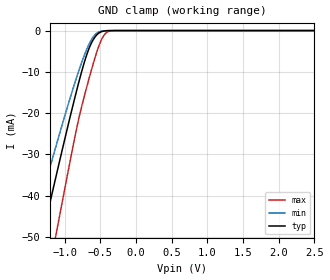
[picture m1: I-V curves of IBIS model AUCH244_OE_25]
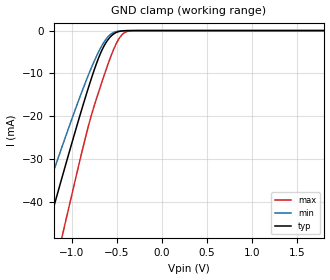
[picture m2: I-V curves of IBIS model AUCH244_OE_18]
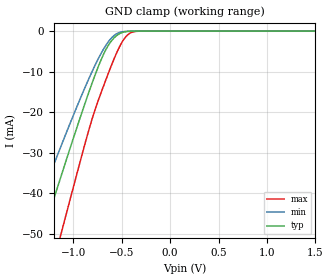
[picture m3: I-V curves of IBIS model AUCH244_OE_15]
| TEXAS INSTRUMENTS INCORPORATED
| Standard Linear and Logic Group
| IBIS Model of SN74AUCH244
| OCTAL BUFFER/DRIVER WITH 3-STATE OUTPUTS
| This file contains package information for the following:
|  QFN 20-pin (RGY) package as [Component] AUCH244_RGY
| This device can be powered at the following Vccs:
|  2.5 volt Vcc
|  1.8 volt Vcc
|  1.5 volt Vcc
|  1.2 volt Vcc
|  0.8 volt Vcc
| This file provides unique models under the [Model Selector] for each Vcc.
| For operation at a specific Vcc, select the appropriate model after each
| [Model Selector] keyword.
[IBIS Ver]   3.2
[Comment char]  |_char
[File Name]   sn74auch244.ibs
[File Rev]   1.1 | x_die
[Date]   October 17, 2002
[Source]   Data created from TI-SPICE simulations at TI-SLL.
[Notes]   The following is an IBIS list for the SN74AUCH244.
   Please contact sllibis@ti.com with questions and
   comments concerning SLL IBIS models.
   -The waveforms for the AUCH244_OUT Pullup and
   Pulldown are caused by the circuitry that helps reduce
   overshoot and undershoot in transmission lines (EMI).
   These waveforms are normal for this particular design.
   -Power-clamp data has been deleted since there is no
   power-clamp diode in the device.
   -Due to presence of bus hold at input, GND-clamp curves
   have non-monotonic warnings.
   -Due to the fact that the device is 5-V input/output
   tolerant, the pullup data has some non-monotonic warnings.
   -End point warning due to AC and DC mismatch.
[Disclaimer] Property of Texas Instruments Incorporated.  Unauthorized
   reproduction and/or distribution is strictly prohibited.
   This product is protected under copyright law.
   Created  2002, (C) Copyright  2002, Texas Instruments
   Incorporated, All Rights Reserved
   UNLESS THERE IS A SIGNED, WRITTEN AGREEMENT TO THE
   CONTRARY, TEXAS INSTRUMENTS (TI) IS PROVIDING THE IBIS
   MODELS  AND WITHOUT ANY WARRANTY, EXPRESSED OR
   IMPLIED.  TI assumes no liability for:
   1) the accuracy of the IBIS models provided to your
   company;
   2) the proper functioning of these IBIS Models in your
   design or for any resulting applications; or
   3) infringement of patents, copyrights or intellectual
   property rights resulting from your use of these IBIS
   models.
   TI provides IBIS Models as a service to our customers.
   You and your company shall not distribute, sell or give
   these models to anyone else without prior written
   permission from TI.
   TI reserves the right to make changes to our products or
   to discontinue any semiconductor product or service
   without notice, and advises our customers to obtain the
   latest version of relevant information to verify, before
   placing orders, that the information being relied on is
   current.
   Please be aware that your receipt and use of the IBIS
   information provided shall serve as acceptance of these
   terms and conditions.  If you do not accept these terms,
   you should return or destroy the IBIS models and any
   other accompanying information immediately.
| Component AUCH244_RGY 20-pin QFN
[Component]   AUCH244_RGY
[Manufacturer]   Texas Instruments, Inc.
[Package]
|   typ   min   max
R_pkg   0.046   0.035   0.058
L_pkg   1.131nH   0.880nH   1.396nH
C_pkg   0.165pF   0.142pF   0.175pF
[Pin]   signal_name   model_name   R_pin   L_pin   C_pin
1   1NOE   AUCH244_OE   0.053   1.289nH   0.142pF
2   1A1   AUCH244_IN   0.058   1.386nH   0.172pF
3   2Y4   AUCH244_OUT   0.046   1.111nH   0.173pF
4   1A2   AUCH244_IN   0.039   0.965nH   0.161pF
5   2Y3   AUCH244_OUT   0.035   0.881nH   0.165pF
6   1A3   AUCH244_IN   0.035   0.880nH   0.165pF
7   2Y2   AUCH244_OUT   0.039   0.961nH   0.161pF
8   1A4   AUCH244_IN   0.045   1.105nH   0.172pF
9   2Y1   AUCH244_OUT   0.058   1.386nH   0.172pF
10   GND   GND   0.056   1.352nH   0.159pF
11   2A1   AUCH244_IN   0.053   1.287nH   0.155pF
12   1Y4   AUCH244_OUT   0.058   1.396nH   0.172pF
13   2A2   AUCH244_IN   0.047   1.129nH   0.175pF
14   1Y3   AUCH244_OUT   0.040   0.976nH   0.164pF
15   2A3   AUCH244_IN   0.035   0.884nH   0.169pF
16   1Y2   AUCH244_OUT   0.035   0.881nH   0.168pF
17   2A4   AUCH244_IN   0.039   0.967nH   0.162pF
18   1Y1   AUCH244_OUT   0.046   1.118nH   0.174pF
19   2NOE   AUCH244_OE   0.058   1.396nH   0.175pF
20   VCC   POWER   0.052   1.276nH   0.144pF
| Model AUCH244_OE
[Model Selector]   AUCH244_OE
AUCH244_OE_25   2.5 volt Vcc
AUCH244_OE_18   1.8 volt Vcc
AUCH244_OE_15   1.5 volt Vcc
AUCH244_OE_12   1.2 volt Vcc
AUCH244_OE_08   0.8 volt Vcc
| Model AUCH244_IN
[Model Selector]   AUCH244_IN
AUCH244_IN_25   2.5 volt Vcc
AUCH244_IN_18   1.8 volt Vcc
AUCH244_IN_15   1.5 volt Vcc
AUCH244_IN_12   1.2 volt Vcc
AUCH244_IN_08   0.8 volt Vcc
| Model AUCH244_OUT
[Model Selector]   AUCH244_OUT
AUCH244_OUT_25   2.5 volt Vcc
AUCH244_OUT_18   1.8 volt Vcc
AUCH244_OUT_15   1.5 volt Vcc
AUCH244_OUT_12   1.2 volt Vcc
AUCH244_OUT_08   0.8 volt Vcc
| Models and submodels in the file (15): AUCH244_OE_25 (Input), AUCH244_OE_18 (Input), AUCH244_OE_15 (Input), AUCH244_OE_12 (Input), AUCH244_OE_08 (Input), AUCH244_IN_25 (Input), AUCH244_IN_18 (Input), AUCH244_IN_15 (Input), AUCH244_IN_12 (Input), AUCH244_IN_08 (Input), AUCH244_OUT_25 (3-state), AUCH244_OUT_18 (3-state), AUCH244_OUT_15 (3-state), AUCH244_OUT_12 (3-state), AUCH244_OUT_08 (3-state)
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[Model]   AUCH244_OE_25
Model_type  Input
Vinl=0.7
Vinh=1.7
| variable   typ   min   max
C_comp   2.45pF   1.96pF   2.85pF
[Temperature Range]   40   100   -40
| Ambient temperature   25   85   -40
[Voltage range]   2.5   2.3   2.7
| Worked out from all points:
|   GND clamp passes 1 mA (typ) near -0.55 V on its own axis
[GND Clamp]
| AUCH244_OE_25
|   Voltage   I(typ)   I(min)   I(max)
-3.6V     -226.6mA   -190.3mA   -271.8mA
-1.455V   -60.71mA   -48.79mA   -79.87mA
-1.295V   -48.52mA   -38.74mA   -65.35mA
-1.105V   -34.25mA   -27.09mA   -48.1mA
-850mV    -15.85mA   -12.35mA   -25.34mA
-785mV    -11.51mA   -8.949mA   -20.15mA
-725mV    -7.81mA    -6.074mA   -16.01mA
-625mV    -3.071mA   -2.25mA    -9.633mA
-520mV    -618.6uA   -332uA     -3.783mA
-430mV    -73.2uA    -35.47uA   -776.9uA
-325mV    -3.339uA   -2.035uA   -30.74uA
2.5V      313.9pA    402pA      470.4pA
[Model]   AUCH244_OE_18
Model_type  Input
Vinl=0.5775
Vinh=1.2675
| variable   typ   min   max
C_comp   2.51pF   2.05pF   2.87pF
[Temperature Range]   40   100   -40
| Ambient temperature   25   85   -40
[Voltage range]   1.8   1.65   1.95
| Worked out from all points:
|   GND clamp passes 1 mA (typ) near -0.55 V on its own axis
[GND Clamp]
| AUCH244_OE_18
|   Voltage   I(typ)   I(min)   I(max)
-3.6V     -226.6mA   -190.3mA   -271.8mA
-1.435V   -59.19mA   -47.53mA   -78.05mA
-1.26V    -45.87mA   -36.57mA   -62.17mA
-1.105V   -34.25mA   -27.09mA   -48.1mA
-1.08V    -32.4mA    -25.59mA   -45.83mA
-810mV    -13.15mA   -10.23mA   -22.06mA
-685mV    -5.638mA   -4.364mA   -13.41mA
-565mV    -1.378mA   -858.8uA   -6.102mA
-490mV    -325.9uA   -162.9uA   -2.495mA
-425mV    -63.96uA   -31.11uA   -688.8uA
-300mV    -1.501uA   -1.001uA   -11.88uA
1.8V      203.2pA    298.4pA    235.5pA
[Model]   AUCH244_OE_15
Model_type  Input
Vinl=0.49
Vinh=1.04
| variable   typ   min   max
C_comp   2.54pF   2.10pF   2.92pF
[Temperature Range]   40   100   -40
| Ambient temperature   25   85   -40
[Voltage range]   1.5   1.4   1.6
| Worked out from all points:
|   GND clamp passes 1 mA (typ) near -0.55 V on its own axis
[GND Clamp]
| AUCH244_OE_15
|   Voltage   I(typ)   I(min)   I(max)
-3.6V     -226.6mA   -190.3mA   -271.8mA
-1.465V   -61.48mA   -49.43mA   -80.77mA
-1.29V    -48.15mA   -38.43mA   -64.9mA
-1.13V    -36.11mA   -28.6mA    -50.37mA
-1.08V    -32.4mA    -25.59mA   -45.83mA
-815mV    -13.48mA   -10.49mA   -22.45mA
-695mV    -6.152mA   -4.773mA   -14.06mA
-575mV    -1.605mA   -1.034mA   -6.664mA
-500mV    -407.2uA   -207.5uA   -2.896mA
-435mV    -83.64uA   -40.42uA   -873uA
-310mV    -2.072uA   -1.331uA   -17.49uA
1.5V      165.9pA    259.7pA    172.1pA
